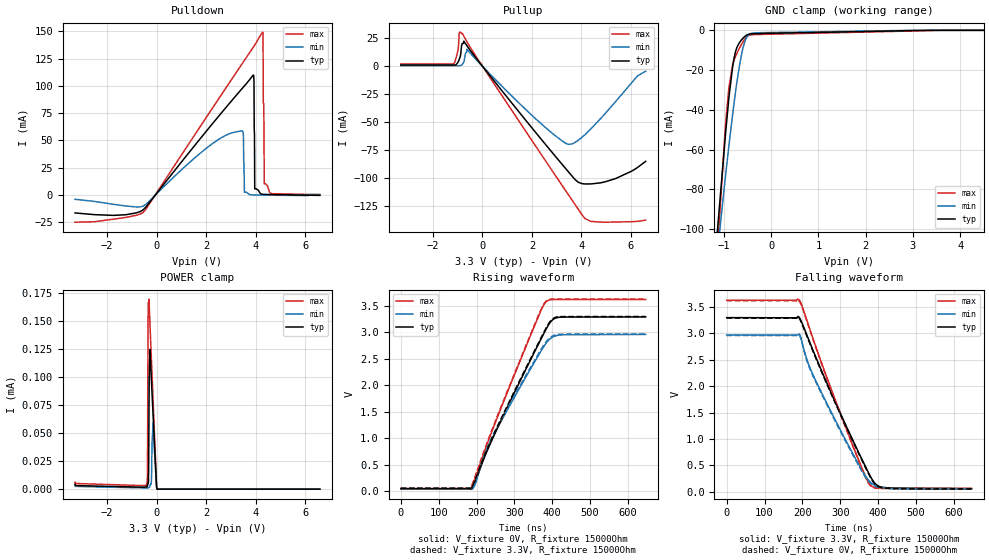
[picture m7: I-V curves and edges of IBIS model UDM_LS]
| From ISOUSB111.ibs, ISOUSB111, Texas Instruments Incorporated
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[Model]   UDM_LS
Model_type   I/O
Polarity   Non-Inverting
Enable   Active-Low
Vinl = 0.8
Vinh = 2
Vmeas = 1.65
Vref = 1.65
Cref = 7pF
Rref = 15000
|   typ   min   max
C_comp   8pF   5pF   10pF
[Voltage Range]   3.3   2.97   3.63
[Temperature Range]   27   150   -40
[Pullup Reference]   3.3   2.97   3.63
[Pulldown Reference]   -0   -0   0
[Power Clamp Reference]   3.3   2.97   3.63
[GND Clamp Reference]   0   0   0
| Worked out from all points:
|   slope of the pulldown table from 0 to 0.495 V, typ, clamps not added: 34.8 ohm
|   slope of the pullup table from 0 to 0.495 V, typ, clamps not added: 35.9 ohm
|   falling waveform, V_fixture 3.3V, R_fixture 15000Ohm: 20-80 % time 121ns typ, 122ns min, 112ns max; typ from 3.3 V to 0.057 V
|   rising waveform, V_fixture 0V, R_fixture 15000Ohm: 20-80 % time 130ns typ, 130ns min, 119ns max; typ from 0.05 V to 3.29 V
|   rising waveform, V_fixture 3.3V, R_fixture 15000Ohm: 20-80 % time 130ns typ, 129ns min, 119ns max; typ from 0.057 V to 3.3 V
|   falling waveform, V_fixture 0V, R_fixture 15000Ohm: 20-80 % time 121ns typ, 121ns min, 112ns max; typ from 3.29 V to 0.05 V
[Pulldown]
|   Voltage   I(typ)   I(min)   I(max)
-3.3V     -16.47mA   -3.956mA   -24.95mA
-537.9mV  -13.47mA   -10.11mA   -15.82mA
3.452V    97.49mA    58.83mA    120.2mA
3.551V    100.1mA    2.347mA    123.5mA
3.907V    109.9mA    72.33uA    135.5mA
3.937V    104.4mA    61.93uA    136.5mA
3.967V    5.559mA    51.57uA    137.5mA
4.283V    625.1uA    -56.97uA   149.4mA
4.303V    541.5uA    -63.61uA   148.4mA
4.313V    537.7uA    -66.93uA   84.38mA
4.353V    520.6uA    -80.16uA   10.24mA
6.6V      -359.4uA   452.5uA    311.4uA
[GND Clamp]
|   Voltage   I(typ)   I(min)   I(max)
-3.3V     -1.288A    -1.121A    -1.582A
-1.3V     -147.2mA   -148.5mA   -173mA
-973.5mV  -54.43mA   -74.96mA   -50.1mA
-894.3mV  -33.89mA   -58.12mA   -28.9mA
-815.1mV  -18.32mA   -42.37mA   -17.26mA
-785.4mV  -14.06mA   -36.77mA   -15.01mA
-735.9mV  -9.387mA   -27.92mA   -12.19mA
-627mV    -4.804mA   -12.27mA   -7.027mA
-567.6mV  -3.283mA   -6.365mA   -4.739mA
-498.3mV  -2.185mA   -2.858mA   -2.96mA
-240.9mV  -1.597mA   -1.202mA   -2.075mA
6.6V      0A         0A         0A
[Pullup]
|   Voltage   I(typ)   I(min)   I(max)
-3.3V     1.143mA    463.2uA    2.098mA
-1.181V   1.062mA    442.5uA    1.977mA
-993.3mV  3.478mA    442.1uA    14.1mA
-933.9mV  6.461mA    535.6uA    30.2mA
-815.1mV  20.51mA    1.633mA    29.48mA
-627mV    18.34mA    15.2mA     22.01mA
1.957V    -54.01mA   -43.06mA   -65.11mA
3.491V    -94.97mA   -69.95mA   -115.6mA
3.868V    -103.8mA   -66.36mA   -127.9mA
4.382V    -105.4mA   -56.14mA   -139mA
5.392V    -100.5mA   -31.47mA   -139.6mA
6.6V      -85.16mA   -4.422mA   -137.9mA
[POWER Clamp]
|   Voltage   I(typ)   I(min)   I(max)
-3.3V     4.356uA    3.599uA    6.245uA
-409.2mV  1.966uA    1.064uA    3.741uA
-369.6mV  3.036uA    1.032uA    12.57uA
-349.8mV  5.266uA    1.012uA    143.2uA
-330mV    6.515uA    1.302uA    167.3uA
-310.2mV  65.78uA    1.419uA    169.9uA
-300.3mV  97.63uA    1.542uA    164.5uA
-270.6mV  124.9uA    2.821uA    148.2uA
-211.2mV  97.44uA    6.822uA    116.2uA
-151.8mV  70.31uA    59.2uA     84.12uA
16.5mV    0A         0A         0A
6.6V      0A         0A         0A
[Ramp]
R_load = 15000
|   typ   min   max
dV/dt_r   1.94459/1.29827e-07   1.74775/1.29419e-07   2.13997/1.18997e-07
dV/dt_f   1.94482/1.21392e-07   1.74773/1.21538e-07   2.14021/1.11582e-07
[Falling Waveform]
V_fixture = 3.3V
V_fixture_min = 2.97V
V_fixture_max = 3.63V
R_fixture = 15000Ohm
C_fixture = 0F
|   Time   V(typ)   V(min)   V(max)
0s        3.299V     2.969V     3.628V
191.1ns   3.309V     2.987V     3.635V
200.1ns   3.176V     2.802V     3.497V
219ns     2.838V     2.363V     3.094V
253.3ns   2.244V     1.837V     2.385V
356.3ns   627.7mV    418.1mV    463.9mV
375ns     352.6mV    216mV      167.1mV
384.7ns   226.4mV    150.7mV    96.14mV
411.8ns   80.42mV    82.78mV    67.82mV
646.7ns   57.34mV    56.08mV    61.1mV
[Rising Waveform]
V_fixture = 0V
V_fixture_min = 0V
V_fixture_max = 0V
R_fixture = 15000Ohm
C_fixture = 0F
|   Time   V(typ)   V(min)   V(max)
0s        49.96mV    47.57mV    54.35mV
184.3ns   49.98mV    47.61mV    49.68mV
195.1ns   169.5mV    112.9mV    231.2mV
223.7ns   692.3mV    727.5mV    811.1mV
249.7ns   1.111V     1.12V      1.3V
369.6ns   2.865V     2.641V     3.404V
384.7ns   3.074V     2.806V     3.583V
400.7ns   3.236V     2.912V     3.618V
419.8ns   3.286V     2.949V     3.619V
646.7ns   3.291V     2.96V      3.621V
[Rising Waveform]
V_fixture = 3.3V
V_fixture_min = 2.97V
V_fixture_max = 3.63V
R_fixture = 15000Ohm
C_fixture = 0F
|   Time   V(typ)   V(min)   V(max)
0s        57.34mV    56.06mV    61.1mV
184.3ns   57.35mV    56.09mV    56.9mV
195.1ns   193.8mV    133mV      258.8mV
223.7ns   721.5mV    755.3mV    838.5mV
251.5ns   1.169V     1.178V     1.359V
360.9ns   2.765V     2.564V     3.277V
384.7ns   3.095V     2.832V     3.597V
400.7ns   3.254V     2.932V     3.628V
419.8ns   3.297V     2.963V     3.628V
646.7ns   3.299V     2.969V     3.628V
[Falling Waveform]
|Gnd
V_fixture = 0V
V_fixture_min = 0V
V_fixture_max = 0V
R_fixture = 15000Ohm
C_fixture = 0F
|   Time   V(typ)   V(min)   V(max)
0s        3.291V     2.961V     3.621V
191.1ns   3.294V     2.976V     3.619V
215.9ns   2.876V     2.4V       3.145V
249.7ns   2.288V     1.866V     2.442V
334.3ns   942.1mV    683.4mV    844mV
365.8ns   468.4mV    284.7mV    286.6mV
379.6ns   272.9mV    161.3mV    113.4mV
392ns     141mV      103.7mV    69.54mV
411.8ns   70.17mV    72.38mV    60.21mV
646.7ns   49.97mV    47.59mV    54.35mV
